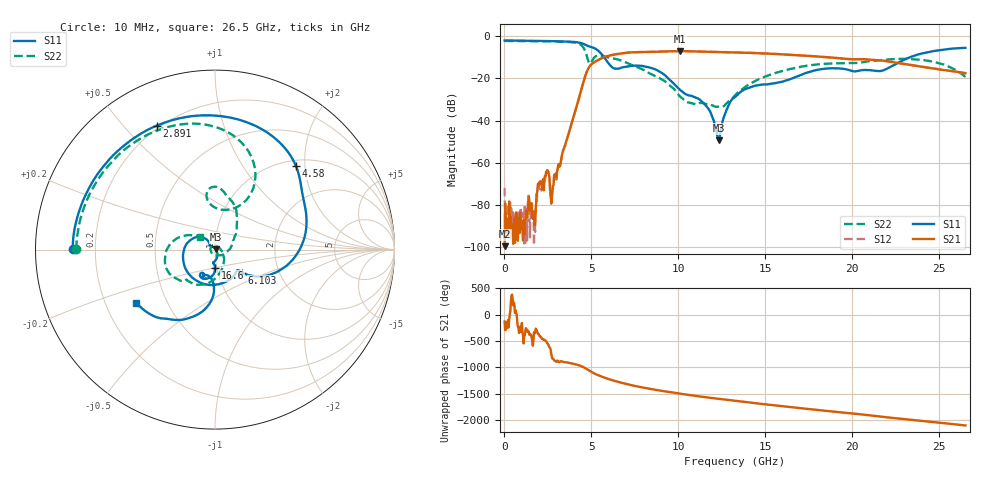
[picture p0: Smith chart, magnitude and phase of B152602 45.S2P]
!  2-Port S-parameters saved by WinCal
! VAR MeasName=S-Parameters (CALIBRATED_DATA) read from VNA (N5242A)
! VAR MeasDate=2016-1-5 16:32:36
! VAR NAME=B152602 45
! VAR FILENAME=B152602 45.S2P
! VAR DATE=2016-1-5 16:32:37
! VAR PHYS_PORTS=1,2
# Hz S DB R 50
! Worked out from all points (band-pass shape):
!   801 points, 10 MHz to 26.5 GHz, reference 50 ohm
!   highest |S21| = -7.07 dB at 10.11 GHz (marker M1); lowest = -99.5 dB at 10 MHz (marker M2)
!   |S21| within 3 dB of the highest: 5.694 GHz to 18.76 GHz (13.06 GHz wide, 107 % of centre)
!   lowest |S11| = -49.3 dB at 12.33 GHz (marker M3), VSWR 1.01, Z = 50.3 + j0.195 ohm
!   |S11| at or under -10 dB: 5.732 GHz to 23.31 GHz (17.57 GHz wide, 121 % of centre)
!   |S22| runs from -33.5 to -2.2 dB; largest |S21 - S12| = 0.0024
!   S11 on the Smith chart (normalised r, x): 10 MHz: 0.12, +0.00; 2.891 GHz: 0.19, +0.62; 4.58 GHz: 1.12, +1.80; 6.103 GHz: 1.30, -0.35; 16.6 GHz: 0.98, -0.20; 26.5 GHz: 0.33, -0.27
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1e7  -2.01 179.7  -99.50 -131.1  -71.82 25.3  -2.24 179.8
1.755625e8  -2.02 176.4  -88.19 108.9  -87.76 23.4  -2.24 177.3
1.665625e9  -2.20 145.4  -83.11 -134.0  -83.68 82.6  -2.36 153.9
2.427212e9  -2.29 127.7  -64.65 -160.7  -64.38 -163.7  -2.44 140.5
2.692112e9  -2.31 120.8  -79.34 -22.2  -77.25 -31.2  -2.46 135.4
2.890788e9  -2.34 115.2  -66.54 -153.4  -67.56 -152.6  -2.49 131.2
4.447075e9  -3.36 53.3  -24.49 98.3  -24.49 98.4  -4.45 73.9
4.579525e9  -3.77 45.8  -20.67 77.7  -20.68 77.7  -5.93 63.9
5.142438e9  -5.56 15.0  -12.44 -32.8  -12.44 -32.7  -10.30 99.0
6.1027e9  -14.02 -40.4  -9.05 -154.1  -9.04 -154.0  -10.28 77.4
7.394088e9  -13.98 -102.1  -7.61 95.1  -7.60 95.2  -13.86 52.6
8.851038e9  -16.45 161.0  -7.33 5.0  -7.32 4.8  -19.48 21.3
1.010931e10  -25.52 129.7  -7.07 -60.4  -7.08 -60.4  -28.69 -60.4
1.159938e10  -33.07 131.2  -7.34 -128.0  -7.34 -128.0  -32.16 147.7
1.232785e10  -49.26 34.3  -7.47 -158.2  -7.46 -158.2  -33.32 72.0
1.3255e10  -28.75 -70.7  -7.66 165.1  -7.66 165.1  -28.01 -13.9
1.487751e10  -22.92 -97.3  -8.17 103.5  -8.14 103.4  -19.55 -66.2
1.659936e10  -19.77 -89.7  -8.91 41.2  -8.87 41.3  -15.26 -94.6
1.769208e10  -16.51 -96.6  -9.45 2.9  -9.42 3.1  -13.66 -110.0
2.020862e10  -16.63 -115.9  -10.96 -80.8  -10.91 -80.8  -12.73 -133.7
2.209604e10  -14.92 -93.8  -11.99 -150.9  -11.93 -151.0  -11.01 -148.9
2.65e10  -5.52 -146.0  -17.54 58.6  -17.54 58.2  -19.33 139.8
